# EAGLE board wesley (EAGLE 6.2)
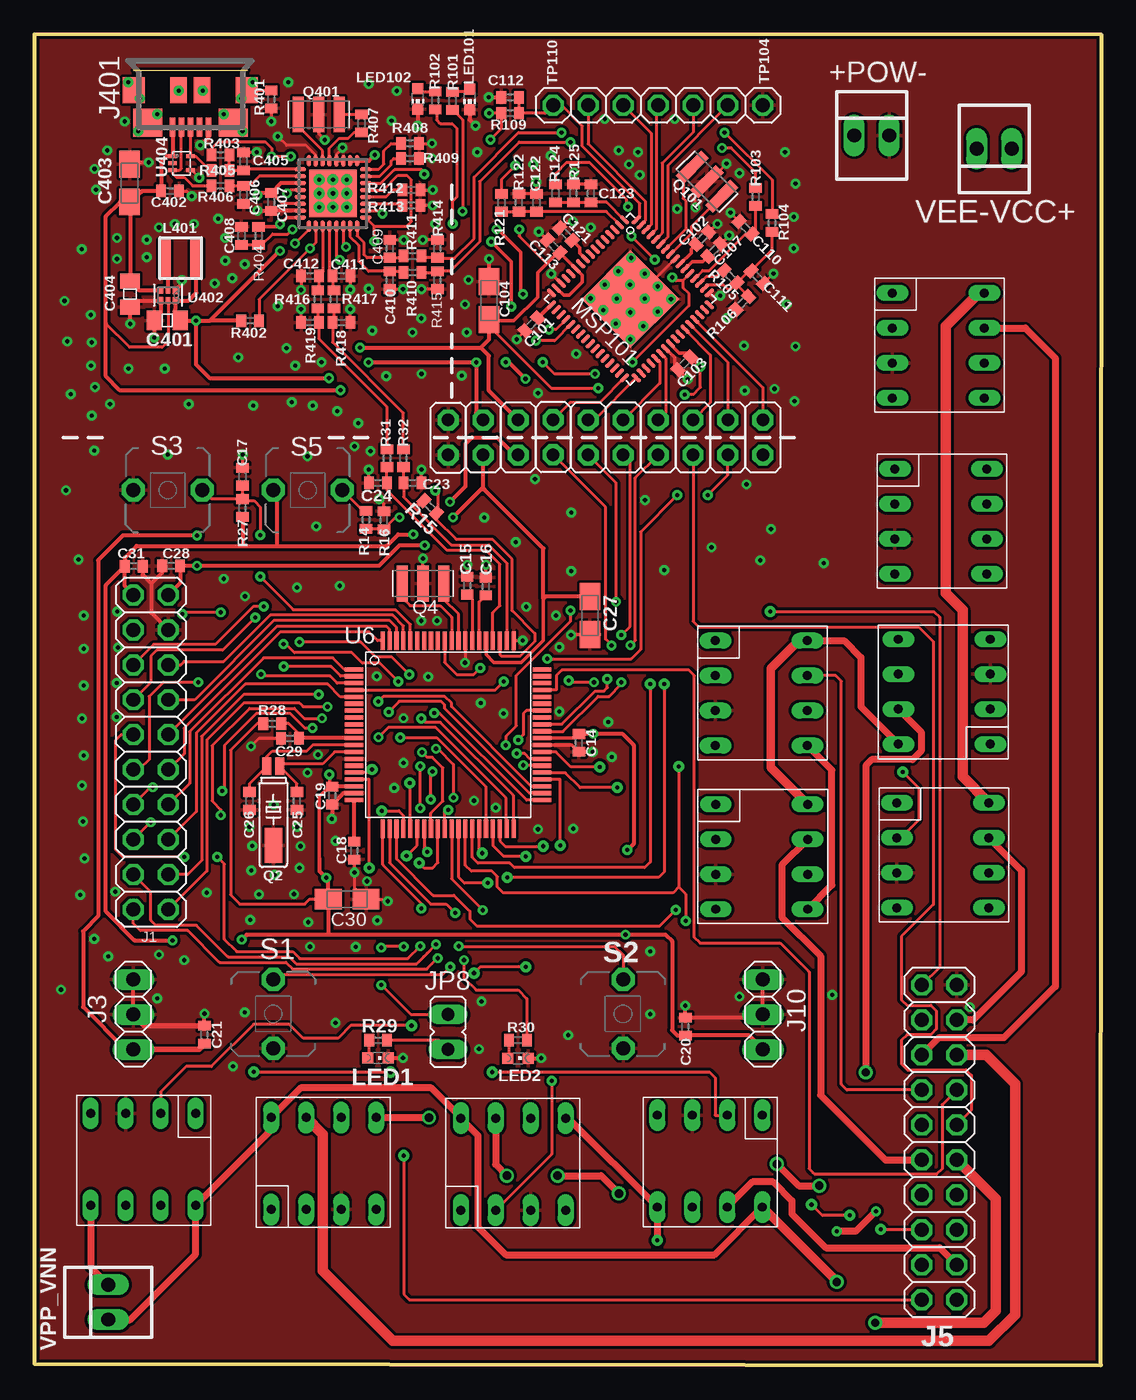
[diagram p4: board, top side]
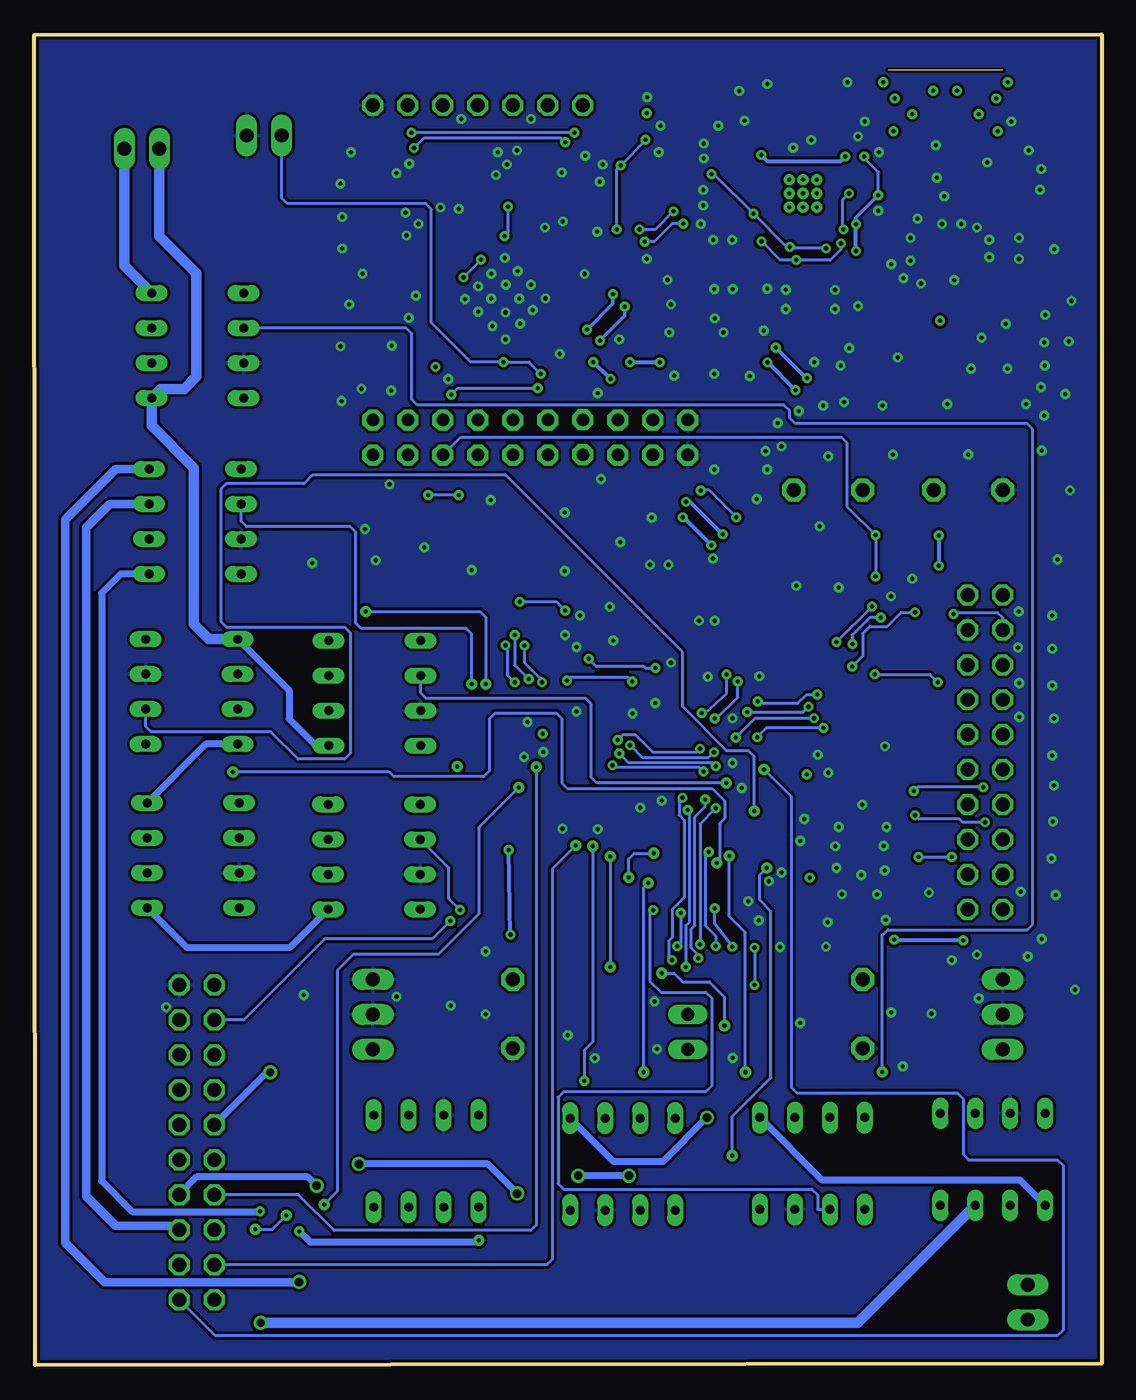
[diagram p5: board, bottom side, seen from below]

Size 77.5 x 96.67 mm. Coordinates in mm from the lower left corner, seen from the top.
Outline: 0,96.67 0,0.1 77.44,0 77.5,96.65 0,96.67
Copper layers (1*16): Top 0.0178mm / dielectric 12mil / Bottom 0.0178mm
Design rules: minimum track width 6mil, minimum drill 12mil, track to track 6mil, track to pad 6mil, pad to pad 6mil, via to via 8mil, smd to smd 6mil, copper to edge 8mil, drill to drill 8mil, minimum pad ring 10mil, minimum via ring 8mil, stop-mask expansion 8mil, vias tented up to drill 15mil, thermal gap 8mil
Net classes: 0 Default: width 0.203 mm, drill 0.305 mm, clearance 0.152 mm; 1 Ground: width 0.203 mm, drill 0.305 mm, clearance 0.152 mm to class 0, clearance 0.152 mm; 2 Power: width 0.203 mm, drill 0.305 mm, clearance 0.152 mm to class 0, clearance 0.152 mm to class 1, clearance 0.152 mm

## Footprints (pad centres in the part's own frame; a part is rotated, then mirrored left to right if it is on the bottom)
22-23-2021 = drill 1 long: 1 -1.27,0; 2 1.27,0
C0402 = smd 0.7 x 0.9: 1 -0.65,0; 2 0.65,0
A/3216-18R = smd 1.95 x 1.5: + 1.375,0; - -1.375,0
CSMD0805 = smd 1.092 x 1.397: 1 -0.94,0; 2 0.94,0
RHB_S-PQFP-N32 = smd 0.85 x 0.3: 1 -2.375,1.75; 2 -2.375,1.25; 3 -2.375,0.75; 4 -2.375,0.25; 5 -2.375,-0.25; 6 -2.375,-0.75; 7 -2.375,-1.25; 8 -2.375,-1.75; 17 2.375,-1.75; 18 2.375,-1.25; 19 2.375,-0.75; 20 2.375,-0.25; 21 2.375,0.25; 22 2.375,0.75; 23 2.375,1.25; 24 2.375,1.75 | smd 0.3 x 0.85: 9 -1.75,-2.375; 10 -1.25,-2.375; 11 -0.75,-2.375; 12 -0.25,-2.375; 13 0.25,-2.375; 14 0.75,-2.375; 15 1.25,-2.375; 16 1.75,-2.375; 25 1.75,2.375; 26 1.25,2.375; 27 0.75,2.375; 28 0.25,2.375; 29 -0.25,2.375; 30 -0.75,2.375; 31 -1.25,2.375; 32 -1.75,2.375 | smd 3.45 x 3.45: EXP 0,0 | drill 0.3 pad 0.6: EXP@1 -1,1; EXP@2 0,1; EXP@3 1,1; EXP@4 -1,0; EXP@5 0,0; EXP@6 1,0; EXP@7 -1,-1; EXP@8 0,-1; EXP@9 1,-1
2X10 = drill 1.016 octagon: 1 -11.43,-1.27; 2 -11.43,1.27; 3 -8.89,-1.27; 4 -8.89,1.27; 5 -6.35,-1.27; 6 -6.35,1.27; 7 -3.81,-1.27; 8 -3.81,1.27; 9 -1.27,-1.27; 10 -1.27,1.27; 11 1.27,-1.27; 12 1.27,1.27; 13 3.81,-1.27; 14 3.81,1.27; 15 6.35,-1.27; 16 6.35,1.27; 17 8.89,-1.27; 18 8.89,1.27; 19 11.43,-1.27; 20 11.43,1.27
1X03 = drill 1.016 long: 1 -2.54,0; 2 0,0; 3 2.54,0
HIROSE-ZX62R-B-5P = smd 1.35 x 0.4: D+ 2.675,0; D- 2.675,-0.65; GND 2.675,1.3; NC 2.675,0.65; VBUS 2.675,-1.3 | smd 1.9 x 1.6: SHIELD1 0,4.1; SHIELD2 0,-4.1 | smd 2 x 2.1: SHIELD3 2.35,3.1; SHIELD4 2.35,-3.1 | smd 1.9 x 1.2: SHIELD5 0,0.85; SHIELD6 0,-0.85
JP1M = drill 0.914 pad 1.524 octagon: 1 0,-1.27; 2 0,1.27
JP1 = drill 0.914 long: 1 0,-1.27; 2 0,1.27
L-NR3010 = smd 0.9 x 2.7: P$1 -1.15,0; P$2 1.15,0
CHIPLED_0603@1 = smd 0.8 x 0.8: A 0,-0.75; C 0,0.75
CHIP-LED0603 = smd 0.8 x 0.8: A 0,-0.75; C 0,0.75
RGC64 = smd 0.825 x 0.28: 1 -4.36,3.75; 2 -4.36,3.25; 3 -4.36,2.75; 4 -4.36,2.25; 5 -4.36,1.75; 6 -4.36,1.25; 7 -4.36,0.75; 8 -4.36,0.25; 9 -4.36,-0.25; 10 -4.36,-0.75; 11 -4.36,-1.25; 12 -4.36,-1.75; 13 -4.36,-2.25; 14 -4.36,-2.75; 15 -4.36,-3.25; 16 -4.36,-3.75; 33 4.36,-3.75; 34 4.36,-3.25; 35 4.36,-2.75; 36 4.36,-2.25; 37 4.36,-1.75; 38 4.36,-1.25; 39 4.36,-0.75; 40 4.36,-0.25; 41 4.36,0.25; 42 4.36,0.75; 43 4.36,1.25; 44 4.36,1.75; 45 4.36,2.25; 46 4.36,2.75; 47 4.36,3.25; 48 4.36,3.75 | smd 0.28 x 0.825: 17 -3.75,-4.36; 18 -3.25,-4.36; 19 -2.75,-4.36; 20 -2.25,-4.36; 21 -1.75,-4.36; 22 -1.25,-4.36; 23 -0.75,-4.36; 24 -0.25,-4.36; 25 0.25,-4.36; 26 0.75,-4.36; 27 1.25,-4.36; 28 1.75,-4.36; 29 2.25,-4.36; 30 2.75,-4.36; 31 3.25,-4.36; 32 3.75,-4.36; 49 3.75,4.36; 50 3.25,4.36; 51 2.75,4.36; 52 2.25,4.36; 53 1.75,4.36; 54 1.25,4.36; 55 0.75,4.36; 56 0.25,4.36; 57 -0.25,4.36; 58 -0.75,4.36; 59 -1.25,4.36; 60 -1.75,4.36; 61 -2.25,4.36; 62 -2.75,4.36; 63 -3.25,4.36; 64 -3.75,4.36 | smd 5 x 5: TP 0,0
8-DIP = drill 0.65 long: 1 3.81,3.81; 2 1.27,3.81; 3 -1.27,3.81; 4 -3.81,3.81; 5 -3.81,-2.87; 6 -1.27,-2.87; 7 1.27,-2.87; 8 3.81,-2.87
MS3V-T1R = smd 0.635 x 1.27: P1 -0.47,-4.43; P2 0.47,-4.43 | smd 1.27 x 2.54: P3 0,1.3
MURATA-FILTER_CSTCR = smd 0.8 x 2.6: 1 -1.5,0; 2 0,0; 3 1.5,0
R0402 = smd 0.7 x 0.9: 1 -0.65,0; 2 0.65,0
PBTH = drill 1.016 pad 1.676 octagon: 1 -0.001,0.001; 2 5.001,0.001
1X01 = drill 1.016 octagon: 1 0,0
PN80 = smd 1.35 x 0.3: 1 -6.825,4.75; 2 -6.825,4.25; 3 -6.825,3.75; 4 -6.825,3.25; 5 -6.825,2.75; 6 -6.825,2.25; 7 -6.825,1.75; 8 -6.825,1.25; 9 -6.825,0.75; 10 -6.825,0.25; 11 -6.825,-0.25; 12 -6.825,-0.75; 13 -6.825,-1.25; 14 -6.825,-1.75; 15 -6.825,-2.25; 16 -6.825,-2.75; 17 -6.825,-3.25; 18 -6.825,-3.75; 19 -6.825,-4.25; 20 -6.825,-4.75; 41 6.825,-4.75; 42 6.825,-4.25; 43 6.825,-3.75; 44 6.825,-3.25; 45 6.825,-2.75; 46 6.825,-2.25; 47 6.825,-1.75; 48 6.825,-1.25; 49 6.825,-0.75; 50 6.825,-0.25; 51 6.825,0.25; 52 6.825,0.75; 53 6.825,1.25; 54 6.825,1.75; 55 6.825,2.25; 56 6.825,2.75; 57 6.825,3.25; 58 6.825,3.75; 59 6.825,4.25; 60 6.825,4.75 | smd 0.3 x 1.35: 21 -4.75,-6.825; 22 -4.25,-6.825; 23 -3.75,-6.825; 24 -3.25,-6.825; 25 -2.75,-6.825; 26 -2.25,-6.825; 27 -1.75,-6.825; 28 -1.25,-6.825; 29 -0.75,-6.825; 30 -0.25,-6.825; 31 0.25,-6.825; 32 0.75,-6.825; 33 1.25,-6.825; 34 1.75,-6.825; 35 2.25,-6.825; 36 2.75,-6.825; 37 3.25,-6.825; 38 3.75,-6.825; 39 4.25,-6.825; 40 4.75,-6.825; 61 4.75,6.825; 62 4.25,6.825; 63 3.75,6.825; 64 3.25,6.825; 65 2.75,6.825; 66 2.25,6.825; 67 1.75,6.825; 68 1.25,6.825; 69 0.75,6.825; 70 0.25,6.825; 71 -0.25,6.825; 72 -0.75,6.825; 73 -1.25,6.825; 74 -1.75,6.825; 75 -2.25,6.825; 76 -2.75,6.825; 77 -3.25,6.825; 78 -3.75,6.825; 79 -4.25,6.825; 80 -4.75,6.825
DRY6 = smd 0.559 x 0.305: 1 -0.356,0.508 | smd 0.508 x 0.305: 2 -0.381,0; 3 -0.381,-0.508; 4 0.381,-0.508; 5 0.381,0; 6 0.381,0.508
TPD2E001-DRL = smd 0.3 x 0.6: 1 -0.5,-0.65; 2 0,-0.65; 3 0.5,-0.65; 4 0.5,0.65; 5 -0.5,0.65

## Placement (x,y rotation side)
+POW-  22-23-2021  [22-23-2021]  60.81,89.33 0 top
C14  100n  [C0402]  39.54,45.2 270 top
C15  220n  [C0402]  31.43,56.63 90 top
C16  220n  [C0402]  32.78,56.57 90 top
C17  1n  [C0402]  15.11,64.54 90 top
C18  470n  [C0402]  23.23,37.38 90 top
C19  100n  [C0402]  21.63,41.38 90 top
C20  100n  [C0402]  47.27,24.59 90 top
C21  100n  [C0402]  12.34,24 90 top
C23  10p  [C0402]  27.46,64.08 0 top
C24  10p  [C0402]  24.94,64.08 180 top
C25  12p  [C0402]  19.06,40.98 90 top
C26  12p  [C0402]  15.62,40.98 90 top
C27  4u7  [A/3216-18R]  40.34,54.46 90 top
C28  100n  [C0402]  9.93,58.06 0 top
C29  100n  [C0402]  18.57,45.53 180 top
C30  10u  [A/3216-18R]  22.71,33.85 180 top
C31  100n  [C0402]  7.21,58.04 180 top
C101  470n  [C0402]  36.09,75.61 225 top
C102  220n  [C0402]  48.5,81.86 45 top
C103  100n  [C0402]  47.21,72.77 225 top
C104  10u  [A/3216-18R]  33,77.33 270 top
C107  220n  [C0402]  49.36,81 45 top
C110  10p  [C0402]  51.64,82.63 135 top
C111  10p  [C0402]  52.5,79.04 315 top
C112  1n  [C0402]  34.55,92.09 180 top
C113  100n  [C0402]  37.7,81.27 135 top
C121  100n  [C0402]  38.6,82.17 135 top
C122  33p  [C0402]  36.46,84.45 270 top
C123  33p  [C0402]  40.41,85.13 270 top
C401  1u  [CSMD0805]  9.65,75.9 0 top
C402  100n  [C0402]  9.86,85.29 0 top
C403  4u7  [A/3216-18R]  6.91,85.88 270 top
C404  1u  [CSMD0805]  6.95,77.8 90 top
C405  22p  [C0402]  15.19,87.45 90 top
C406  22p  [C0402]  15.19,85.01 270 top
C407  100n  [C0402]  17.2,84.51 270 top
C408  100n  [C0402]  15.04,82.04 90 top
C409  22p  [C0402]  25.81,81.1 90 top
C410  22p  [C0402]  25.81,78.82 270 top
C411  22p  [C0402]  22.3,79.12 0 top
C412  22p  [C0402]  20.02,79.12 180 top
IC401  TUSB2046BIRHBIRHB  [RHB_S-PQFP-N32]  21.68,85.12 0 top
J1  [2X10]  8.46,44.53 270 top
J3  PWR  [1X03]  7.19,25.48 270 top
J5  [2X10]  65.71,16.18 270 top
J10  PWR  [1X03]  52.91,25.48 270 top
J401  [HIROSE-ZX62R-B-5P]  11.33,92.61 270 top
JP1  +5V  [JP1M]  32.59,67.39 180 top
JP2  +3V3  [JP1M]  35.13,67.39 180 top
JP3  GND  [JP1M]  30.05,67.39 0 top
JP4.1  SBW_TST  [JP1M]  50.37,67.39 180 top
JP4.2  SBW_RST  [JP1M]  47.83,67.39 180 top
JP4.3  SBW_NC  [JP1M]  52.91,67.39 180 top
JP6.1  TXD  [JP1M]  45.29,67.39 180 top
JP6.2  RXD  [JP1M]  42.75,67.39 180 top
JP6.3  CTS  [JP1M]  40.21,67.39 180 top
JP6.4  RTS  [JP1M]  37.67,67.41 180 top
JP8  LED1_PWR  [JP1]  30.05,24.21 180 top
L401  2.2uH (NR3010T2R2M)  [L-NR3010]  10.62,80.42 0 top
LED1  [CHIPLED_0603@1]  24.96,22.31 270 top
LED2  [CHIPLED_0603@1]  35.13,22.29 270 top
LED101  red  [CHIP-LED0603]  31.61,91.95 180 top
LED102  green  [CHIP-LED0603]  27.85,91.97 180 top
MSP101  MSP430F5528IRGC  [RGC64]  43.28,77.46 315 top
OPTO1  VO3150A  [8-DIP]  53.29,36.93 90 top
OPTO2  VO3150A  [8-DIP]  65.61,48.92 270 top
OPTO3  VO3150A  [8-DIP]  53.26,48.82 90 top
OPTO4  VO3150A  [8-DIP]  66.12,74.07 90 top
OPTO5  VO3150A  [8-DIP]  66.45,37.03 90 top
OPTO6  VO3150A  [8-DIP]  21.01,15.11 180 top
OPTO7  VO3150A  [8-DIP]  7.9,14.48 0 top
OPTO8  VO3150A  [8-DIP]  34.77,15.06 180 top
OPTO9  VO3150A  [8-DIP]  66.29,61.29 90 top
OPTO10  VO3150A  [8-DIP]  49.05,14.35 0 top
Q2  32.768kHz  [MS3V-T1R]  17.35,39.07 180 top
Q4  CSTCR4M00G15L99  [MURATA-FILTER_CSTCR]  28.22,56.78 0 top
Q101  PIEZO_CSTCR4M00G15L99  [MURATA-FILTER_CSTCR]  48.84,85.98 135 top
Q401  CSTCR6M00G15L99  [MURATA-FILTER_CSTCR]  20.65,90.86 0 top
R14  100R  [R0402]  24.08,61.4 270 top
R15  1k4  [R0402]  28.74,62.34 135 top
R16  1M  [R0402]  25.37,61.38 270 top
R27  47k  [R0402]  15.1,62.27 270 top
R28  0R  [R0402]  17.27,46.6 180 top
R29  470R  [R0402]  24.97,23.6 180 top
R30  470R  [R0402]  35.12,23.61 180 top
R31  27R  [R0402]  25.6,65.89 270 top
R32  27R  [R0402]  26.8,65.89 270 top
R101  470  [R0402]  30.37,91.85 270 top
R102  390  [R0402]  29.11,91.87 270 top
R103  27R  [R0402]  52.37,84.86 270 top
R104  27R  [R0402]  53.57,82.98 270 top
R105  1k4  [R0402]  50.55,79.07 135 top
R106  1M  [R0402]  51.41,77.17 45 top
R109  47k  [R0402]  34.55,90.94 180 top
R121  220k  [R0402]  33.92,84.44 270 top
R122  220k  [R0402]  35.18,84.44 90 top
R124  240k  [R0402]  37.85,85.13 270 top
R125  150k  [R0402]  39.14,85.13 90 top
R401  33R  [R0402]  17.2,91.95 270 top
R402  10k  [R0402]  15.67,75.87 0 top
R403  1k5  [R0402]  13.51,87.91 0 top
R404  47k  [R0402]  16.28,82.04 270 top
R405  22R  [R0402]  13.51,86.79 180 top
R406  22R  [R0402]  13.51,85.67 180 top
R407  1k5  [R0402]  23.75,90.2 270 top
R408  15k  [R0402]  27.28,88.75 180 top
R409  15k  [R0402]  27.28,87.66 180 top
R410  22R  [R0402]  27.46,79.38 0 top
R411  22R  [R0402]  27.46,80.57 0 top
R412  15k  [R0402]  27.38,85.37 180 top
R413  15k  [R0402]  27.38,84.25 180 top
R414  15k  [R0402]  29.26,81.1 90 top
R415  15k  [R0402]  29.26,78.82 270 top
R416  22R  [R0402]  20.57,77.42 270 top
R417  22R  [R0402]  21.74,77.42 270 top
R418  15k  [R0402]  22.3,75.74 0 top
R419  15k  [R0402]  20.02,75.74 180 top
S1  [PBTH]  17.35,28.02 270 top
S2  [PBTH]  42.75,28.02 270 top
S3  RST  [PBTH]  7.19,63.58 0 top
S5  BSL  [PBTH]  17.35,63.58 0 top
TP104  TEST_PIN2  [1X01]  52.91,91.52 0 top
TP105  TEST_PIN2  [1X01]  50.37,91.52 0 top
TP106  TEST_PIN2  [1X01]  47.83,91.52 0 top
TP107  TEST_PIN2  [1X01]  45.29,91.52 0 top
TP108  TEST_PIN2  [1X01]  42.75,91.52 0 top
TP109  TEST_PIN2  [1X01]  40.21,91.52 0 top
TP110  TEST_PIN2  [1X01]  37.67,91.52 0 top
U6  MSP430F5529IPNR  [PN80]  30.05,45.8 0 top
U402  TPS62237DRY  [DRY6]  9.7,77.72 270 top
U404  TPD2E001DRLR  [TPD2E001-DRL]  10.68,87.31 270 top
VEE-VCC+  22-23-2021  [22-23-2021]  69.7,88.37 180 top
VPP_VNN  22-23-2021  [22-23-2021]  5.36,4.57 90 top

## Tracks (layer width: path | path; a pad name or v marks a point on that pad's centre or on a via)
!OC  (via drill 0.3 pad 0.66)
  Top 0.203: IC401.14 22.43,81.43 v22.63,81.23 | IC401.10 20.43,81.54 v20.02,81.13 16.32,77.43 R402.2 | IC401.18 25.05,83.87 v25.27,83.64 | IC401.22 25.16,85.87 26.14,86.84 28.14,86.84 28.32,86.67 v28.32,86.51
  Bottom 0.203: v20.02,81.13 22.53,81.13 v22.63,81.23 22.86,81.23 v25.27,83.64 28.14,86.51 v28.32,86.51
!PWRON  (via drill 0.3 pad 0.66)
  Top 0.203: IC401.13 21.93,80.54 v22.17,80.29 | v24.69,81.64 24.69,82.73 | 24.69,82.73 IC401.17 24.69,82.73 | IC401.21 25.32,85.37 26.39,86.44 27.05,86.44 27.38,86.11 27.38,83.08 27.03,82.73 24.69,82.73 | IC401.9 19.93,82.49 v18.92,81.48
  Bottom 0.203: v24.69,81.64 23.34,80.29 v22.17,80.29 22.15,80.26 19.71,80.26 18.92,81.05 v18.92,81.48
+3V3  (via drill 0.3, 0.3 pad 0.66)
  Top 0.203: v40.59,45.87 40.61,45.87 | R28.2 16.17,46.6 14.25,44.68 14.25,34.16 14.91,33.5 19.63,33.5 19.99,33.86 21.83,33.86 C30.+ | 21.84,31.32 21.79,31.27
  Top 0.254: U6.50 39.23,45.55 C14.1 40.57,45.85 v40.59,45.87 | C31.2 6.58,58.05 | R27.2 15.11,61.61 | 20.7,36.78 20.7,41.3 21.45,42.05 | 21.65,42.05 21.45,42.05 | 21.45,42.05 21.45,42.87 v21.41,42.9
  Top 0.305: J1.1 6.56,56.58 C31.2 5.18,56.66 5.18,32.94 7.26,30.86 v10.03,30.86 | U6.18 21.65,42.05 C19.2 | 6.58,58.05 6.58,58.67 7.42,59.51 15.11,59.51 | 15.11,59.51 17.6,59.51 | 17.6,59.51 25.58,59.51 26.42,60.35 v27.51,60.35 | 15.11,61.61 15.11,59.51 | S5.1 17.6,63.32 17.6,59.51 | v40.59,45.87 42.67,45.87 43.51,45.03 43.51,37.87 v43.05,37.41 | 21.41,31.27 21.79,31.27 v42.93,31.27 45.85,31.27 46.3,30.81 46.3,24.33 46.69,23.95 47.25,23.95 C20.1 51.91,23.94 J10.3 | 21.41,31.27 15.42,31.27 v15.06,30.91 | 20.7,36.78 20.7,35.89 v21.18,35.41 21.33,35.26 C30.+ 21.33,31.35 21.41,31.27 | v30.18,62.71 31.32,63.86 31.32,66.93 31.78,67.39 33.6,67.39 34.87,66.12 JP2.2
  Bottom 0.305: v27.51,60.35 29.87,62.71 v30.18,62.71 | v10.03,30.86 14.73,30.86 v15.06,30.91 | v42.93,31.27 v43.05,37.41
+5V  (via drill 0.3 pad 0.66)
  Top 0.254: U6.65 32.8,51.61 33.38,51.03 35.36,51.03 36.96,52.63 36.96,55.68 37.11,55.83
  Top 0.305: J1.2 10.58,56.81 C28.2 v11.81,58.06 25.02,58.06 26.52,59.56 v28.35,59.56 | 36.96,55.68 36.96,59.33 32.68,63.61 32.49,63.61 32.36,63.55 | C27.+ 37.11,55.83 | v11.81,60.27 6.43,60.27 4.62,58.47 4.62,32.61 3.53,31.52 3.53,26.01 6.6,22.94 J3.3 | 12.61,23.35 C21.1 | v30.4,61.6 32.36,63.55 | 32.36,63.55 32.59,63.78 JP1.2
  Top 0.406: J3.3 11.93,22.94 C21.1
  Bottom 0.254: 30.38,61.6 v30.4,61.6
  Bottom 0.305: v28.35,59.56 30.38,61.6 | v11.81,60.27 v11.81,58.06
AVCC
  Top 0.203: C29.1 19.22,45.86 18.47,46.61 17.94,46.61 R28.1
  Top 0.305: U6.11 19.23,45.55 C29.1
EZFET_AVBUS
  Top 0.203: R124.2 | R124.2 R125.1 | R125.1 | R125.1 C123.2 41.56,84.48 MSP101.1
EZFET_AVCCOUT2ADC
  Top 0.203: R121.2 | R121.2 R122.1 C122.2 | C122.2 36.88,83.79 | MSP101.2 41.54,83.8 C122.2
EZFET_LED0  (via drill 0.3 pad 0.66)
  Top 0.203: R101.2 31.09,90.47 v31.09,83.82 | MSP101.20 37.88,75.24 v37.36,75.24
  Top 0.254: v33.55,82.5 33.68,82.5 35.33,80.85 35.33,77.95 v35.48,77.8
  Bottom 0.203: v31.09,83.82 32.41,82.5 v33.55,82.5
  Bottom 0.254: v35.48,77.8 35.48,77.11 v37.36,75.24
EZFET_LED1  (via drill 0.3 pad 0.66)
  Top 0.203: R102.2 29.21,91.12 29.21,90.48 29.49,90.2 30.33,90.2 30.66,89.87 30.66,84.84 30.38,84.56 v30.38,82.93 | MSP101.21 37.77,74.42 v36.42,74.42
  Top 0.254: v34.62,76.89 34.62,80.16 v33.17,81.61
  Bottom 0.203: v33.17,81.61 32.49,81.61 31.17,82.93 v30.38,82.93
  Bottom 0.254: v36.42,74.42 34.62,76.23 v34.62,76.89
EZFET_PU.0/DP
  Top 0.203: MSP101.50 48.91,78.49 50.04,78.49 50.34,78.18 50.57,78.18 R105.1 | R105.1 51.9,79.5 C111.1 53.57,81.03 R104.2 | R106.2 51.01,78.49 R105.1
EZFET_PU.1/DM
  Top 0.203: MSP101.52 48.53,79.53 49,79.53 51.64,82.17 C110.1 52.38,82.44 R103.2
EZFET_PUR
  Top 0.203: MSP101.51 48.81,79.1 49.56,79.1 49.99,79.53 R105.2
EZFET_RST
  Top 0.203: MSP101.64 43.97,83.45 43.97,84.38 39.8,88.54 39.8,90.02 38.3,91.52 TP110.1 37.1,90.95 R109.1 C112.1
EZFET_SBW_NC
  Top 0.203: MSP101.45 52.91,71.02 JP4.3.1
EZFET_SBW_RST
  Top 0.203: MSP101.43 47.25,75.23 49.1,73.38 49.1,69.93 JP4.2.1
EZFET_SBW_TST
  Top 0.203: MSP101.44 50.37,72.85 JP4.1.1
EZFET_TCK
  Top 0.203: MSP101.63 44.37,83.15 44.37,84.56 40.21,88.72 TP109.1
EZFET_TDI
  Top 0.203: MSP101.61 45.19,82.54 45.19,91.41 TP107.1
EZFET_TDO
  Top 0.203: MSP101.60 45.59,82.24 45.59,87.33 47.83,89.56 TP106.1
EZFET_TEST
  Top 0.203: MSP101.59 46,81.94 46,87.15 TP105.1
EZFET_TMS
  Top 0.203: MSP101.62 44.78,82.85 44.78,89.48 TP108.1
EZFET_UARTCTS
  Top 0.203: MSP101.32 41.05,69.93 38.91,69.93 JP6.4.1
EZFET_UARTRTS
  Top 0.203: MSP101.33 40.65,68.66 JP6.3.1
EZFET_UARTRXD
  Top 0.203: MSP101.38 45.51,73.49 45.85,73.15 45.85,69.22 JP6.1.1
EZFET_UARTTXD
  Top 0.203: MSP101.37 45.42,72.85 45.42,71.32 JP6.2.1
EZFET_V18
  Top 0.254: MSP101.55 46.91,80.01 47.7,80.8 47.7,81.06 C102.1
EZFET_VBUS  (via drill 0.3 pad 0.66)
  Top 0.203: R124.1 37.85,86.56 38.66,87.38 40.31,87.38 42.98,84.71 42.98,84.28 v43.1,84.15 | MSP101.53 47.6,79.28 47.09,78.77 | 47.09,78.77 46.58,78.77 v46.33,79.02 | v43.36,82.02 v45.06,80.32 | 47.09,78.77 47.09,78.28 47.55,77.83 47.55,76.96 47.52,76.96 v43.43,72.87 | v40.72,72.01 37.77,72.01 v36.91,72.87 | J401.VBUS | 9.7,75.01 U402.5 9.7,74.37 9.27,73.94 6.91,73.94 5.18,75.67
  Top 0.305: v22.23,70.84 6.17,70.84 5.18,71.83 5.18,75.67 5.18,83.46 6.22,84.5 C403.+ | v24.26,72.85 v32.08,72.85 32.08,69.16 JP1.1 | v34.24,72.87 34.44,72.87 v35.66,71.65 | C403.+ 7.83,85.29 C402.1 9.2,85.43 9.2,87.4 9.61,87.81 U404.1 J401.VBUS | U402.3 7.58,78.11 C404.2 6.95,84.46 C403.+
  Bottom 0.203: v43.1,84.15 43.1,82.3 43.36,82.04 | 43.36,82.04 v43.36,82.02 | 45.06,80.29 v45.06,80.32 46.33,79.05 v46.33,79.02 | v40.72,72.01 41.58,72.87 v43.43,72.87 45.82,72.87 48.67,75.72 48.67,83.97 49.07,84.38 59.13,84.38 59.54,84.79 +POW-.1 | 43.33,82.04 43.36,82.04
  Bottom 0.305: v22.23,70.84 24.23,72.85 v24.26,72.85 | v35.66,71.65 35.69,71.65 v36.91,72.87 | v34.24,72.87 32.08,72.87 v32.08,72.85
EZFET_VCC  (via drill 0.3 pad 0.66)
  Top 0.203: v33.02,90.96 33.89,90.96 R109.2 33.9,89.81 v33.12,89.03 | v47.22,70.51 47.83,70.51 48.36,71.04 v48.36,72.52 | C104.+ 33.06,75.45 37.54,70.97 v40.95,70.97 | R121.1 33.92,86.14 v34.93,87.15 | v35.2,82.5 35.2,82.02 37.21,80.01 | v18.62,87.81 v17.22,87.81 17.22,88.42 16.76,88.87 13.34,88.87 12.86,88.4 R403.1 | IC401.6 17.99,84.37 C407.1
  Top 0.254: MSP101.15 37.91,78.24 38.43,77.72 38.84,77.72 39.78,78.66 39.78,79.19 MSP101.11 C113.1 38.01,80.81 37.21,80.01 36.55,79.35 36.55,77.6 34.82,75.87 33.09,75.87 C104.+ | v48.36,72.52 47.67,73.21 C103.1 47.36,73.53 46.84,73.53 46.19,74.18 MSP101.40 | IC401.8 18.32,83.37 v17.83,82.88 17.64,82.69 R404.1
  Top 0.305: 21.37,71.69 v21.39,71.7 12.73,71.7 11.74,72.7 v11.74,75.87 | v23.65,73.91 32.41,73.91 | C104.+ 33,74.5 32.41,73.91 | 32.41,73.91 33,73.32 33,70.78 JP2.1 | L401.P$2 11.77,77.91 11.2,77.34 U402.6 10.21,76.68 10.21,76.28 C401.2 10.62,75.87 v11.74,75.87 | IC401.25 IC401.26 24.3,87.49 v24.71,87.91 | v11.74,75.87 12.75,75.87 | 12.75,75.87 v17.83,80.95 | IC401.3 17.91,85.87 C407.1 16.37,85.16 v16.21,84.99 | R402.1 12.75,75.87
  Bottom 0.203: v47.22,70.51 46.76,70.97 v40.95,70.97 | v33.12,89.03 33.12,88.95 v34.93,87.15 35.2,86.87 v35.2,82.5 | v16.21,84.99 16.21,86.67 17.22,87.68 v17.22,87.81
  Bottom 0.254: v17.83,82.88 17.83,83.36 v16.21,84.99
  Bottom 0.305: v21.39,71.7 21.44,71.7 v23.65,73.91 | v24.71,87.91 24.28,87.48 18.95,87.48 v18.62,87.81 | v17.83,80.95 v17.83,82.88
EZFET_VREF
  Top 0.254: MSP101.9 39.6,80.8 39.6,81.17 C121.1
EZFET_VUSB
  Top 0.254: MSP101.54 47.27,79.66 47.78,80.16 48.53,80.16 C107.1
EZFET_XT2IN
  Top 0.203: MSP101.57 47.73,82.25 47.73,82.74 Q101.1
EZFET_XT2OUT
  Top 0.203: MSP101.58 47.32,82.55 47.32,84.56 47.12,84.76 47.12,86.37 Q101.3
GND  (via drill 0.3 pad 0.66)
  Top 0.203: C405.2 15.99,88.1 v16.15,88.11 | C412.2 v19.37,78.12 v19.36,78.11 | C411.2 22.95,78.15 v22.94,78.13 | R418.2 22.95,76.69 v22.94,76.71 | R419.2 19.37,76.62 v19.36,76.71 | U6.61 v35.46,52.63 | C16.2 32.82,57.25 v32.79,58.14 | C15.2 31.45,57.29 v31.45,58.14 | U6.68 31.3,51.06 v31.27,51.03 | Q4.2 v28.22,58.6 | C24.2 24.29,64.81 v24.28,65.05 | C23.2 28.11,64.81 v28.12,65.05 | R16.1 25.37,62.59 v25.04,62.92 | C17.2 15.14,65.22 v15.14,66.14 | C18.1 23.23,35.98 v23.24,35.79 23.24,34.69 C30.- 25.51,33.85 v25.65,33.71 | C110.2 50.67,83.59 v50.55,83.72 | C111.2 53.59,79.22 v53.67,79.3 | MSP101.49 49.21,77.7 v49.81,77.7 | R106.1 v50.32,76.07 | 38.23,82.63 38.68,83.08 v39.12,83.08 | C123.1 R125.2 39.19,85.83 v39.19,86.64 | 35.2,85.12 R122.2 C122.1 36.47,85.89 v36.45,85.98 | C101.2 35.03,74.55 v35.03,74.52 | MSP101.56 44.91,78.74 | v50.27,87.27 48.97,85.98 Q101.2 48.01,85.14 v48.01,84.1 | R408.1 v28.88,88.75 | R409.1 v28.88,87.66 | R413.1 v28.93,84.25 | R412.1 v28.93,85.37 | C409.2 26.81,81.75 v26.82,81.74 | R414.2 28.21,81.75 v28.19,81.74 | R415.2 v28.13,78.17 v28.12,78.16 | C410.2 v26.76,78.17 v26.77,78.16 | R401.2 v17.2,90.35 | IC401.27 IC401.28 21.93,87.94 v22.38,88.44 | Q401.2 20.65,89.48 v21.08,89 | C29.2 16.29,45.53 v15.72,44.96 | C402.2 11.05,85.29 v11.43,84.91 | IC401.31 20.43,87.9 19.71,88.62 18.31,88.62 v17.68,89.26 | 11.38,86.81 11.41,86.81 v11.96,86.26
  Top 0.254: MSP101.14 38.25,78.61 v37.54,79.27 | C121.2 38.23,82.63 | C113.2 37.24,81.76 v36.63,82.35 | v47.45,71.63 46.76,72.31 C103.2 46.51,72.55 46.51,73.18 MSP101.39 | C107.2 49.86,81.46 v50.47,82.07 | C102.2 49.02,82.32 v49.61,82.91 | C27.- 39.01,53.08 v38.96,53.04 | U6.49 39.04,45.05 C14.2 40.51,44.55 v40.54,44.55
  Top 0.305: U404.4 11.38,86.81 | J401.GND 12.63,89.18 v12.04,88.62 | C403.- 7.03,87.38 v8.31,87.38 | U402.1 10.67,78.54 v10.69,78.82 | v8.71,74.65 C401.1 9.2,76.38 U402.4 7.43,77.34 C404.1 6.96,76.85 v6.96,75.64 | C104.- 33.02,78.22 v33.02,80.37 | LED102.C v27.85,90.05 v27.84,90.04 | LED101.C 31.61,90.46 v32.03,90.04 | C112.2 v33,92.09 v32.99,92.1 | C31.1 7.86,57.41 8.48,56.79 | 8.48,56.79 8.48,54.66 J1.4 | C28.1 9.28,57.59 8.48,56.79 | J10.1 J10.2 52.67,25.24 C20.2 v47.27,26.11 | C21.2 v12.34,25.53 | J3.2 J3.1 | LED1.C 26.76,22.31 v26.77,22.33 | LED2.C 36.77,22.29 36.78,22.3 v36.8,22.3 | U6.19 22.45,41.55 C19.1 21.63,39.71 v21.59,39.68 | v16.21,83.87 C407.2 IC401.7 | v45.26,78.36 45.03,78.36 44.37,79.02 44.63,79.02 44.91,78.74
  Top 0.406: C21.2 8.01,24.65 J3.2
  other vias: 19.08,39.09 15.62,39.09 43.33,80.44 40.39,77.5 42.21,75.67 46.23,77.44 44.32,79.3 42.39,79.48 41.43,78.49 43.26,78.49 42.29,77.47 41.3,76.63 43.28,74.52 44.22,75.49 45.26,76.53 44.32,77.47 43.28,76.48 46.69,84 3.2,58.52 2.29,63.55 4.17,68.99 9.68,66.14 19.84,66.01 20.47,60.93 15.29,55.85 19.08,56.49 22.17,56.62 29.24,54.08 24.87,50.04 28.6,50.01 26.8,46.99 41.94,44.17 34.06,47.35 35.71,55.09 32.66,61.57 36.35,64.36 67.92,26.01 52.71,58.47 38.13,52.17 38.99,61.93 38.99,57.68 45.75,57.76 44.35,62.84 51.71,63.98 49.17,59.41 55.19,70.03 51.54,74.07 55.27,74.02 54.64,77.06 55.14,81.13 55.27,85.83 54.51,88.11 55.14,83.41 51.21,86.59 43.97,86.46 43.84,88.11 42.44,88.24 37.49,87.86 36.22,87.22 40.41,82.65 43.18,87.22 41.43,90.53 46.51,90.53 26.31,92.56 25.93,90.4 29.11,82.91 31.27,77.06 32.16,88.11 31.52,78.84 27.46,75.03 28.09,76.05 24.28,78.21 24.54,75.16 28.12,72.01 25.55,71.86 51.59,70.79 22,69.32 23.52,68.43 31.39,75.03 24.41,66.4 23.24,66.75 20.22,69.7 18.69,69.95 18.95,72.62 20.85,72.87 18.31,73.89 17.68,76.94 15.27,79.98 14.38,78.97 13.11,78.59 13.87,80.24 13.87,81.89 13.36,83.29 11.58,82.91 10.19,82.91 9.04,82.65 8.15,81.76 8.15,80.49 24.28,93.07 18.44,93.19 5.99,81.89 5.99,80.37 6.55,90.35 2.39,74.37 2.18,77.32 5.28,88.24 4.37,86.89 2.64,70.54 3.43,81.08 4.47,85.39 4.09,76.3 4.17,74.3 4.11,72.62 4.39,71.04 5.49,69.82 11.2,69.82 15.9,69.7 3.58,54.46 4.34,66.45 3.58,52.04 3.58,49.38 3.45,46.96 3.58,44.3 3.45,42.11 3.53,39.5 3.63,36.8 3.33,34.16 4.34,30.96 5.36,29.69 10.87,29.41 23.34,30.38 51.21,26.77 38.13,47.47 41.68,46.71 39.14,38.96 32.41,48.11 31.93,41 53.49,60.73 24.89,32.31 33.5,40.49 26.14,41.94 26.8,43.74 36.58,38.94 21.87,38.07 24.16,35.15 18.85,34.21 21.87,24.87 14.43,21.69 32.28,22.96 38.76,23.98 32.46,26.42 44.73,25.5 13.74,57.12 57.94,26.9 1.93,27.28 17.45,35.61 15.75,35.94 19.25,36.12 19.33,37.69 17.37,40.72 15.82,37.72 19.84,43.03 28.09,54.08 6.07,52.12 34.95,59.79 37.87,54.46 20.02,30.4 44.73,30.05 36.58,70.61 39.34,73.46 53.75,70.92 31.04,71.88 57.33,58.27 6.02,54.74 5.97,49.56 5.97,47.09 15.67,32.33 12.52,34.32 5.87,34.39 20.6,44.35 16.31,34.19 19.89,32.18 6.83,72.39 9.47,72.39 14.81,73.2 8.92,26.64 15.27,25.63 9.04,29.82
  pour Top (isolate 0.203, rank 2): -1.96,98.53 -1.83,-1.32 78.94,-1.85 78.69,98.35
  pour Bottom (isolate 0.203, rank 2): -2.41,98.93 -1.93,-1.7 79.1,-1.4 78.82,98.53
  pour Top (isolate 0.203): 24.23,45.54 15.44,45.54 14.66,44.78 14.63,35.92 15.54,34.95 19.28,34.95 20.22,35.86 20.22,42.67 21.59,44.04 24.23,44.04
  pour Top (isolate 0.203): 23.27,92.07 22.5,92.84 18.92,92.84 18.26,92.18 18.26,89.38 20.02,87.07 22.48,87.02 22.91,88.47 22.91,88.67 24.49,88.67 24.49,92.13
  pour Top (isolate 0.203): 31.32,51.64 31.34,54.94 30.76,55.52 30.73,58.06 29.97,58.83 26.39,58.83 25.73,58.17 25.73,55.37 26.47,54.64 29.46,54.64 29.77,54.33 29.77,51.64
HUB_DM1
  Top 0.203: R416.2 20.57,75.83 R419.1 20.67,74.56 25.6,69.62 R31.1
HUB_DM2  (via drill 0.3 pad 0.66)
  Top 0.203: R103.1 52.4,85.54 52.4,86.64 50.62,88.42 v49.94,88.42 | v38.94,88.85 35.2,88.85 32.33,85.98 32.33,81.61 30.19,79.47 R415.1 29.17,79.38 R410.2
  Bottom 0.203: v49.94,88.42 49.23,89.13 39.22,89.13 v38.94,88.85
HUB_DP1
  Top 0.203: R417.2 21.74,75.83 R418.1 21.65,74.31 26.8,69.16 R32.1
HUB_DP2  (via drill 0.3 pad 0.66)
  Top 0.203: R104.1 53.57,86.11 50.14,89.54 v50.11,89.54 | v38.28,89.54 35.15,89.54 31.93,86.31 31.93,81.84 30.51,80.42 29.3,80.42 R414.1 28.22,80.45 R411.2
  Bottom 0.203: v38.28,89.54 v50.11,89.54
N$1
  Top 0.203: 30.41,92.45 R101.1 31.41,92.5 LED101.A
N$2
  Top 0.203: LED102.A 27.9,92.52 R102.1
N$3
  Top 0.203: IC401.15 22.91,82.72 22.91,81.99 23.55,81.36 23.55,80.19 24.27,79.47 C410.1 26.72,79.47 R410.1
N$4
  Top 0.203: R14.1 23.87,62.05 S5.2
N$5
  Top 0.203: R403.2 R405.1 15.18,86.79 C405.1 15.25,86.87 IC401.1
N$6
  Top 0.203: IC401.30 20.93,88.22 19.15,89.99 Q401.1
N$7
  Top 0.203: R29.1 29.39,23.6 JP8.2
N$8
  Top 0.305: MSP101.17 36.57,76.05 C101.1
N$9  (via drill 0.3 pad 0.3)
  other vias: 7.54,89.64
N$10
  Top 0.203: R401.1 15.44,92.6 J401.SHIELD1
N$11
  Top 0.203: R406.1 C406.1 15.33,85.8 15.75,85.8 16.31,86.37 IC401.2
N$12
  Top 0.203: J401.D+ U404.5 11.73,87.81 12.75,86.79 R405.2
N$13
  Top 0.203: J401.D- 10.67,89.92 10.67,86.94 10.54,86.81 U404.3 10.03,86.57 10.31,86.28 10.87,86.28 11.48,85.67 R406.2
N$14
  Top 0.305: U402.2 9.7,79.3 9.47,79.53 L401.P$1
N$15
  Top 0.203: R407.2 23.2,89.55 22.78,89.13 22.15,89.13 21.43,88.41 IC401.29
N$16
  Top 0.203: IC401.11 20.93,79.39 C412.1 20.67,78.16 R416.1
N$17
  Top 0.203: IC401.12 21.43,79.34 C411.1 21.65,78.16 R417.1
N$18
  Top 0.203: IC401.16 23.44,82.73 23.44,82.04 23.95,81.53 23.95,80.67 24.17,80.45 C409.1 26.69,80.45 R411.1
N$19  (via drill 0.3 pad 0.66)
  Top 0.203: IC401.4 18.59,85.37 v18.34,85.12 | C408.1 R404.2 16.52,81.39 17.3,82.17 18.42,82.17 v18.75,82.5
  Bottom 0.203: v18.34,85.12 18.82,84.63 18.82,82.58 v18.75,82.5
N$20
  Top 0.203: R412.2 26.04,85.37 25.53,84.86 IC401.20
N$21
  Top 0.203: IC401.24 24.99,86.87 25.37,87.25 25.37,88.21 25.91,88.75 R408.2
N$22
  Top 0.203: IC401.23 25.08,86.37 25.91,87.2 25.91,87.48 26.09,87.66 R409.2
N$23
  Top 0.203: IC401.19 26.59,84.37 R413.2
N$24  (via drill 0.3 pad 0.3)
  other vias: 8.92,90.88
N$25  (via drill 0.3 pad 0.3)
  other vias: 13.74,90.88
N$26  (via drill 0.3 pad 0.3)
  other vias: 15.11,89.64
N$27  (via drill 0.3 pad 0.3)
  other vias: 15.85,93.19
N$28
  Top 0.203: R407.1 22.16,90.85 Q401.3
N$29  (via drill 0.3 pad 0.3)
  other vias: 15.01,92.02
N$30  (via drill 0.3 pad 0.3)
  other vias: 7.65,92.02
N$31  (via drill 0.3 pad 0.3)
  other vias: 6.81,93.19
N$32
  Top 0.203: LED1.A 24.32,22.43 R29.2
N$33  (via drill 0.3 pad 0.3)
  other vias: 10.49,92.58
N$34  (via drill 0.3 pad 0.3)
  other vias: 12.22,92.58
N$35
  Top 0.203: LED2.A 34.47,22.38 R30.2
P1.0  (via drill 0.3 pad 0.3)
  Top 0.203: U6.21 25.3,36.35 28.09,33.55 v28.09,33.17 | U6.21 | v25.2,27.61 27.33,25.48 JP8.1 | v26.82,30.4 25.27,30.4 v25.2,30.33
  Bottom 0.203: v25.2,30.33 v25.2,27.61 | v26.82,30.4 28.09,32.06 v28.09,33.17
P1.1  (via drill 0.3)
  Top 0.203: U6.22 25.8,36.48 28.78,33.5 29.9,33.5 v30.56,32.84 | v30.81,30.43 42.11,30.43 42.75,29.79 S2.1
  Bottom 0.203: v30.56,32.84 30.56,30.68 v30.81,30.43
P1.2  (via drill 0.3)
  Top 0.203: v46.58,33.07 45.39,31.88 32.16,31.88 31.62,32.41 31.62,32.97 30.45,34.14 28.93,34.14 26.3,36.77 U6.23
  Bottom 0.203: v46.58,33.07 47.4,33.88 47.4,36.12 OPTO1.2
P1.3  (via drill 0.3 pad 0.81)
  Top 0.203: v25.22,40.26 26.47,40.26 26.8,39.93 U6.24
  Bottom 0.203: v25.22,40.26 25.22,44.22 25.63,44.63 27.23,44.63 30.43,47.83 30.43,51.79 43.28,64.64 57.3,64.64 57.91,64.03 63.55,64.03 63.96,63.63 63.96,54.03 63.55,53.62 54.97,53.62 54.56,53.21 54.56,44.42 54.97,44.02 58.34,44.02 60.33,46 69.01,46 69.42,46.41 OPTO2.2
P1.4  (via drill 0.3 pad 0.81)
  Top 0.203: v27.25,42.29 27.25,39.41 27.3,39.37 U6.25
  Bottom 0.203: v27.25,42.29 36.65,42.29 37.06,42.7 37.06,48.03 37.47,48.44 49.05,48.44 49.45,48.84 OPTO3.2
P1.5  (via drill 0.3 pad 0.81)
  Top 0.203: v15.93,21.31 25.83,21.31 v25.86,21.29 | v27.03,36.98 27.8,37.76 U6.26
  Bottom 0.203: v25.86,21.29 25.86,31.42 27.03,32.59 v27.03,36.98 | v15.93,21.31 15.93,31.22 15.52,31.62 5.41,31.62 5,32.03 5,68 5.41,68.4 22.25,68.4 22.66,68.81 22.66,69.34 23.06,69.75 49.68,69.75 50.09,70.16 50.09,74.93 50.5,75.34 OPTO4.2
P1.6  (via drill 0.3)
  Top 0.203: U6.27 28.3,37.51 v28.52,37.29 | 27.76,30.18 v28.02,30.43 27.13,29.54 19.25,29.54 18.75,30.05 14.68,30.05 13.79,30.94 13.79,36.4 v13.28,36.91 | v10.87,36.91 6.43,36.91 5.92,37.41 5.92,45.42 6.3,45.8 J1.9
  Bottom 0.203: v13.28,36.91 v10.87,36.91 | v28.52,37.29 28.78,37.03 28.78,31.95 28.02,31.19 v28.02,30.43
P1.7  (via drill 0.3)
  Top 0.203: U6.28 28.8,40.1 29.67,40.97 29.67,43.38 28.91,44.15 28.52,44.15 v28.14,44.53 | v38.94,54.81 38.94,54.05 35,50.11 35,46.43 34.24,45.67 v34.24,45.03 | v42.24,55.45 42.24,64.08 JP6.3.2
  Bottom 0.203: v38.94,54.81 39.57,55.45 v42.24,55.45 | v28.14,44.53 28.52,44.15 33.35,44.15 v34.24,45.03
P2.0  (via drill 0.3 pad 0.81)
  Top 0.203: U6.29 29.3,36.51 28.88,36.09 28.32,36.09 v27.94,36.47 | v63.07,43.08 64.21,41.94 64.21,39.6 62.92,38.3 OPTO5.2
  Bottom 0.203: v63.07,43.08 | v27.94,36.47 27.74,36.68 27.74,39.34 27.36,39.73 27.36,40.97 28.27,41.88 38.79,41.88 39.19,42.29 39.19,46.96 39.6,47.37 44.04,47.37 44.44,46.96 44.44,43.19 44.88,42.75 51.38,42.75 51.71,43.08 v63.07,43.08
P2.1  (via drill 0.3, 0.3 pad 0.66)
  Top 0.203: U6.30 29.79,40.16 29.97,40.34 v30.05,40.34 | S1.1 17.53,28.02 17.91,28.4 29.67,28.4 v30.2,28.93
  Bottom 0.203: v30.05,40.34 29.92,40.21 29.92,32.21 30.18,31.95 30.18,28.96 v30.2,28.93
P2.2  (via drill 0.3)
  Top 0.203: U6.31 30.3,35.34 32.56,33.07 v32.56,33.05
  Bottom 0.203: OPTO6.2 20.63,11.3 20.63,12.37 21.03,12.78 39.07,12.78 39.47,13.18 39.47,19.46 39.07,19.86 28.73,19.86 28.32,20.27 28.32,26.67 28.73,27.08 31.98,27.08 32.79,27.89 32.79,32.82 v32.56,33.05
P2.3  (via drill 0.3 pad 0.81)
  Top 0.203: v32.92,35.03 31.22,35.03 30.8,35.45 U6.32 | OPTO10.2 49.43,18.16 49.43,20.88 49.02,21.29 v33.25,21.29
  Bottom 0.203: v33.25,21.29 33.25,34.7 v32.92,35.03
P2.4  (via drill 0.3, 0.3 pad 0.81)
  Top 0.203: v46.79,43.49 46.79,34.72 | 46.79,34.72 46.38,34.32 34.04,34.32 33.63,34.72 33.63,35.48 33.22,35.89 31.72,35.89 31.3,36.32 U6.33 | 46.79,34.72 47.3,34.21 v47.3,32.26
  Bottom 0.203: v47.3,32.26 48.59,30.96 56.41,30.96 62.31,25.07 J5.3
P2.5  (via drill 0.3 pad 0.81)
  Top 0.203: v44.73,49.48 44.73,36.55 44.32,36.14 34.85,36.14 34.52,36.47 32.21,36.47 31.8,36.88 U6.34 | v53.44,54.74 65.33,54.74 65.74,54.33 65.74,28.91 J5.1
  Bottom 0.203: v53.44,54.74 45.14,54.74 44.73,54.33 v44.73,49.48
P2.6  (via drill 0.3 pad 0.81)
  Top 0.203: v32.51,37.19 32.51,37.49 32.3,37.49 U6.35 | v45.75,49.48 45.75,35.84 45.34,35.43 v34.34,35.43
  Bottom 0.203: v34.34,35.43 34.34,36.78 33.93,37.19 v32.51,37.19 | v45.75,49.48 45.75,53.11 46.15,53.52 53.75,53.52 54.15,53.92 54.15,60.5 54.56,60.91 62.08,60.91 62.48,61.32 OPTO9.2
P2.7  (via drill 0.3 pad 0.66)
  Top 0.203: 32.79,38.98 U6.36 32.8,42.01 29.21,45.59 v26.57,45.59 | v13.54,39.95 13.54,40.34 12.9,41 12.9,45.01 15.62,47.7 18.87,47.7 19.58,46.99 v20.88,46.99 | v8.46,39.45 J1.15
  Bottom 0.203: v13.54,39.95 13.28,39.7 10.36,39.7 10.11,39.45 v8.46,39.45 | v20.88,46.99 25.17,46.99 v26.57,45.59
P3.0  (via drill 0.3 pad 0.81)
  Top 0.203: U6.37 33.3,37.75 34.06,36.98 35.66,36.98 v35.69,36.96 | v35.69,28.93 32.39,28.93 v31.93,28.47 | v27.38,24.66 22.96,24.66 22.05,23.75 19.53,23.75 18.52,24.77 15.93,24.77 12.85,21.69 11.02,21.69 9.17,19.84 OPTO7.2
  Bottom 0.203: v35.69,36.96 v35.69,28.93 | v31.93,28.47 31.04,28.47 30.4,27.84 28.47,27.84 27.38,26.75 v27.38,24.66
P3.1  (via drill 0.3, 0.3 pad 0.81)
  Top 0.203: U6.38 33.8,38.08 34.19,37.69 v36.96,37.69 | v37.57,20.65 37.57,15.32 OPTO8.2
  Bottom 0.203: v36.96,37.69 36.96,23.47 37.57,22.86 v37.57,20.65
P3.2  (via drill 0.3 pad 0.66)
  Top 0.203: U6.39 34.26,39.01 34.26,41.2 29.16,46.3 25.68,46.3 v24.99,45.62 | v13.64,41.71 13.79,41.86 13.79,45.01 16.1,47.32 18.59,47.32 19.63,46.28 v20.19,46.28 | v8.59,41.99 8.46,41.99 J1.13
  Bottom 0.203: v8.59,41.99 13.36,41.99 v13.64,41.71 | v20.19,46.28 24.33,46.28 v24.99,45.62
P3.3  (via drill 0.3 pad 0.3, 0.3 pad 0.66)
  Top 0.203: U6.40 34.77,39 34.77,41.4 29.49,46.69 28.37,46.69 v28.09,46.96 | v26.42,49.66 25.07,51 23.83,51 23.06,51.77 18.87,51.77 18.26,52.38 v18.09,52.38 | v16.03,54.31 13.67,51.94 8.89,51.94 8.46,51.51 8.46,49.61 J1.7
  Bottom 0.203: v26.42,49.66 26.42,48.51 27.97,46.96 v28.09,46.96 | v16.03,54.31 16.84,54.31 18.11,53.04 18.11,52.4 v18.09,52.38
P3.4  (via drill 0.3 pad 0.3, 0.3 pad 0.66)
  Top 0.203: U6.41 35.74,41.05 29.41,47.37 v29.03,47.37 | v19.25,52.53 23.7,52.53 24.79,51.44 25.96,51.44 v27.23,50.17 | v16.66,55.12 15.9,55.12 13.13,52.35 8.66,52.35 J1.5
  Bottom 0.203: v27.23,50.17 27.23,48.79 28.78,47.37 v29.03,47.37 | v19.25,52.53 v16.66,55.12
P3.5  (via drill 0.3)
  Top 0.203: U6.42 35.95,41.55 29.79,47.7 29.79,47.96 29.54,48.21 26.49,48.21 v25.73,47.45 | J1.20 12.52,35.89 12.52,45.42 15.19,48.08 19.25,48.08 19.51,47.83 v21.29,47.83
  Bottom 0.203: v25.73,47.45 21.67,47.45 v21.29,47.83
P3.6  (via drill 0.3)
  Top 0.203: U6.43 36.08,42.05 30.3,47.83 30.3,48.08 29.79,48.59 25.35,48.59 v24.97,48.21 | J1.18 11.12,35.64 12.14,36.66 12.14,45.67 15.19,48.72 v20.65,48.72
  Bottom 0.203: v24.97,48.21 24.84,48.08 22.05,48.08 21.41,48.72 v20.65,48.72
P3.7  (via drill 0.3 pad 0.81)
  Top 0.203: v38.18,37.74 38.18,42.55 U6.44
  Bottom 0.203: v38.18,37.74 39.88,36.04 39.88,7.7 40.28,7.29 J5.17
P4.0  (via drill 0.3 pad 0.81)
  Top 0.203: J5.15 61.49,9.83 v61.47,9.86 | v59.21,10.87 57.23,10.87 v56.44,11.66 | v42.32,41.96 39.62,41.96 38.56,43.03 36.89,43.03 U6.45
  Bottom 0.203: v61.47,9.86 60.22,9.86 v59.21,10.87 | v56.44,11.66 56.44,11.68 55.47,12.65 55.47,28.7 54.31,29.87 48.13,29.87 45.19,32.82 45.19,39.09 v42.32,41.96
P4.1  (via drill 0.3 pad 0.66)
  Top 0.203: v28.78,41.1 28.78,42.98 v28.91,43.13 | 28.98,29.26 v29.29,29.57 28.5,28.78 18.75,28.78 18.26,29.26 13.44,29.26 11.13,31.57 7.7,31.57 7.19,32.08 J1.19 | U6.46 35.55,43.55 v35.51,43.59
  Bottom 0.203: v28.91,43.13 29.18,43.41 35.33,43.41 v35.51,43.59 | 28.78,40.72 v28.78,41.1 28.78,40.59 29.54,39.83 29.54,31.95 29.79,31.7 29.79,30.3 29.29,29.79 v29.29,29.57
P4.2  (via drill 0.3)
  Top 0.203: J1.17 8.46,34.37 8.46,32.31 8.82,31.95 11.76,31.95 14.05,29.67 18.49,29.67 19,29.16 27.76,29.16 28.27,29.67 28.52,29.92 v29.16,30.56 | v28.02,40.46 v28.02,43.51 | U6.47 35.99,44.05 35.61,44.43 v35.03,44.43
  Bottom 0.203: v28.02,40.46 29.16,39.32 v29.16,30.56 | v28.02,43.51 28.27,43.76 34.37,43.76 v35.03,44.43
P4.3  (via drill 0.3 pad 0.81)
  Top 0.203: v41.05,43.46 38.96,43.46 37.87,44.55 U6.48
  Bottom 0.203: v41.05,43.46 41.05,10.19 41.45,9.78 55.73,9.78 58.32,12.37 J5.13
P4.4/UCA1TXD  (via drill 0.3)
  Top 0.203: U6.51 36.89,46.03 38.38,46.03 40.95,48.59 41.73,48.59 42.62,49.48 v42.62,49.61 | v43.28,52.3 43.64,52.65 43.64,64.47 JP6.1.2
  Bottom 0.203: v42.62,49.61 43.13,50.11 43.13,52.15 v43.28,52.3
P4.5/UCA1RXD  (via drill 0.3)
  Top 0.203: U6.52 36.89,46.56 38.3,46.56 40.72,48.97 41.35,48.97 41.61,49.23 v41.61,49.84 | v42.62,53.04 43.26,53.67 43.26,65.61 JP6.2.2
  Bottom 0.203: v42.62,53.04 42.62,50.85 v41.61,49.84
P4.7  (via drill 0.3)
  Top 0.203: U6.54 35.74,47.55 35.51,47.32 35.51,45.8 v35.13,45.42 | v31.19,29.41 31.19,28.14 32.08,27.25 35.13,27.25 35.76,26.62 R30.1 | v29.16,44.78 29.29,44.78 30.43,43.64 v30.43,41.22
  Bottom 0.203: v30.43,41.22 30.68,40.97 30.68,39.95 30.3,39.57 30.3,33.99 31.19,33.1 31.19,31.06 31.45,30.81 31.45,29.67 v31.19,29.41 | v29.16,44.78 29.41,44.53 32.59,44.53 33.86,45.8 34.75,45.8 v35.13,45.42
P5.2/XT2IN
  Top 0.203: U6.69 30.8,54.55 29.72,55.63 Q4.3
P5.3/XT2OUT
  Top 0.203: Q4.1 26.72,55.73 27.28,55.17 29.46,55.17 30.3,54.33 U6.70
P5.4/XIN
  Top 0.203: U6.12 20.21,45.05 19.76,44.6 17.27,44.6 16.88,44.21 Q2.P2 15.62,42.24 C26.2
P5.5/XOUT
  Top 0.203: C25.2 19.06,42.25 Q2.P1 | Q2.P1 17.87,43.5 | U6.13 21.79,44.55 20.93,43.69 18.01,43.69 Q2.P1
P6.0
  Top 0.203: U6.77 26.8,53.69 26.01,54.48 17.12,54.48 13.77,51.13 10.87,51.13 10.62,50.88 J1.6
P6.1
  Top 0.203: U6.78 26.3,53.59 25.81,54.08 17.37,54.08 11.63,48.34 J1.8
P6.2
  Top 0.203: U6.79 25.8,53.45 25.58,53.67 17.6,53.67 J1.10
P6.3
  Top 0.203: U6.80 24.93,52.62 24.28,53.26 17.86,53.26 10.87,46.28 10.87,44.4 J1.12
P6.4
  Top 0.203: J1.14 11.28,42.27 11.28,46.03 16.64,51.38 21.67,51.38 22.5,50.55 U6.1
P6.5  (via drill 0.3)
  Top 0.203: v13.54,54.69 10.87,54.69 v10.74,54.56 | U6.2 22.24,50.05 21.54,50.75 v18.11,50.75
  Bottom 0.203: v10.74,54.56 10.62,54.69 7.57,54.69 7.19,54.31 J1.3 | v13.54,54.69 14.55,54.69 15.57,53.67 16.84,53.67 17.35,53.16 17.35,51.51 v18.11,50.75
P6.6  (via drill 0.3, 0.3 pad 0.66)
  Top 0.203: v11.89,49.61 9.36,49.61 8.33,48.58 8.33,44 7.59,43.26 J1.11 | U6.3 21.98,49.55 21.47,50.05 16.59,50.05 v16.46,50.18
  Bottom 0.203: v16.46,50.18 12.46,50.18 v11.89,49.61
P6.7  (via drill 0.3 pad 0.3, 0.3 pad 0.66)
  Top 0.203: U6.4 33.48,49.05 v34.09,49.66 | v41.91,52.27 41.48,52.73 41.48,62.33 JP6.4.2 | v40.64,49.61 38.94,49.61 v38.81,49.73
  Bottom 0.203: v41.91,52.27 41.91,51.05 40.64,49.78 v40.64,49.61 | 34.09,49.63 v34.09,49.66 34.42,49.99 38.56,49.99 v38.81,49.73
P7.0
  Top 0.203: J1.16 11.76,40.21 11.76,45.92 15.32,49.48 21.29,49.48 22.22,48.55 U6.5
P7.4
  Top 0.203: J5.8 65.91,18.92 65.91,14.25 65.51,13.84 56.69,13.84 56.52,14.02 56.29,14.25 56.26,14.28 56.26,28.55 54.15,30.66 48.34,30.66 47.93,31.06 47.93,50.09 47.52,50.5 38.3,50.5 37.9,50.09 37.9,49.05 U6.57
P8.1  (via drill 0.3 pad 0.81)
  Top 0.203: v24.51,43.28 24.28,43.05 U6.16
  Bottom 0.203: v24.51,43.28 22.53,41.3 22.53,20.17 22.12,19.76 10.47,19.76 10.06,19.36 10.06,15.32 9.65,14.91 3.2,14.91 2.79,14.5 2.79,2.54 3.2,2.13 64.36,2.13 J5.20
P8.2  (via drill 0.3 pad 0.81)
  Top 0.203: v24.31,36.12 24.31,42.55 U6.17 | v26.82,15.21 26.82,5.16 27.23,4.75 J5.19
  Bottom 0.203: v26.82,15.21 26.82,18.06 24,20.88 24,32.97 24.82,33.78 24.82,35.61 v24.31,36.12
RST/SBWTDIO  (via drill 0.3 pad 0.66)
  Top 0.203: R27.1 12.85,62.92 S3.2 | U6.76 27.3,53.8 26.21,54.89 18.8,54.89 v16.41,57.28 | R27.1 15.23,62.79 15.95,62.79 16.41,62.33 v16.41,60.3 | C17.1 15.1,63.88 R27.1 | JP4.2.2 47.83,54.03 48.23,53.62 64.21,53.62 65.28,52.55 65.28,33.45 62.97,31.14 62.97,26.54 63.37,26.14 65.1,26.14 65.51,25.73 65.51,24.41 65.1,24 63.37,24 62.97,23.6 62.97,21.87 63.37,21.46 67.64,21.46 68.05,21.06 68.05,18.52 J5.10
  Bottom 0.203: v16.41,57.28 v16.41,60.3 18.49,62.38 18.49,67.01 18.9,67.41 46.53,67.41 JP4.2.2
TARGET_DM
  Top 0.203: U6.64 33.3,54.66 33.81,55.17 33.81,58.19 32.82,59.18 29.97,59.18 25.59,63.56 C24.1 R31.2
TARGET_DP
  Top 0.203: 34.26,52.66 U6.62 34.3,58.29 32.99,59.59 30.29,59.59 27.4,62.48 | R32.2 C23.1 26.81,63.07 27.4,62.48 | R15.2 27.95,62.48 27.4,62.48
TARGET_PUR  (via drill 0.3 pad 0.66)
  Top 0.203: U6.63 33.81,52.61 33.81,51.61 33.91,51.51 35.28,51.51 36.35,52.58 36.35,53.16 34.7,54.81 34.7,58.55 33.25,60 30.63,60 29.2,61.43 R15.1 | R14.2 25.35,60.75 R16.2 26.24,61.6 v26.52,61.6 | R15.1 29.13,61.95 | v29.11,63.53 29.34,63.3 29.34,62.02 R15.1
  Bottom 0.203: v26.52,61.6 28.5,63.58 29.06,63.58 v29.11,63.53
TARGET_VUSB
  Top 0.203: U6.66 32.3,55.44 C16.1
TEST/SBWTCK  (via drill 0.3, 0.3 pad 0.66)
  Top 0.203: U6.71 29.8,51.05 30.68,50.17 31.9,50.17 v32.39,50.65 | v37.24,51.31 43.33,51.31 44.02,51.99 44.02,60.53 v46.69,63.2 | v48.9,63.2 50.37,64.67 JP4.1.2
  Bottom 0.203: v37.24,51.31 36.68,50.75 33.22,50.75 33.12,50.65 v32.39,50.65 | v46.69,63.2 v48.9,63.2
V18
  Top 0.203: C15.1 31.8,55.61 U6.67
VCC+
  Top 0.508: OPTO3.8 58.8,52.63 60.02,51.41 60.02,47.83 OPTO2.8
  Top 0.635: OPTO1.8 53.47,43.43 53.47,50.6 55.5,52.63 OPTO3.8
  Top 0.762: OPTO4.8 68.58,77.88 66.19,75.49 66.19,56.08 67.41,54.86 67.41,42.75 OPTO5.8
  Bottom 0.508: OPTO2.8 65.05,45.11 OPTO5.8
  Bottom 0.762: VEE-VCC+.1 70.97,79.86 OPTO4.8
VCORE
  Top 0.305: C18.2 U6.20
VEE-
  Top 0.508: OPTO1.5 57.91,34.87 57.91,43.23 OPTO3.5 | OPTO3.5
  Bottom 0.508: OPTO5.5 66.45,30.35 58.93,30.35 OPTO1.5 | OPTO1.5 | OPTO2.5 59,49 59,46.94 57.07,45.01 OPTO3.5
  Bottom 0.762: VEE-VCC+.2 68.43,82.02 65.74,79.32 65.74,71.81 66.62,70.92 68.33,70.92 OPTO4.5 68.99,68.25 65.91,65.18 65.91,53.82 64.85,52.76 62.76,52.76 OPTO2.5
VNN-  (via drill 0.3, 0.3 pad 0.81, 0.6)
  Top 0.508: OPTO7.5 4.09,7.11 VPP_VNN.2 | OPTO6.5 v28.65,17.98 | v45.24,9.07 OPTO10.5 38.79,17.93 OPTO8.5 | v61.11,11.18 59.66,9.73 v58.27,9.73
  Bottom 0.508: OPTO9.5 71.22,57.48 72.62,56.08 72.62,13.39 70.38,11.15 61.14,11.15 v61.11,11.18 | v45.24,9.07 45.36,8.94 57.48,8.94 v58.27,9.73 | OPTO7.5 5.92,13.44 20.27,13.44 OPTO6.5 | v28.65,17.98 31.85,14.78 35.43,14.78 OPTO8.5
VO1
  Top 0.508: OPTO1.7 54.28,36.32 54.28,32.54 57.1,29.72 57.1,19.61 61.8,14.91 J5.11
VO2  (via drill 0.6)
  Top 0.508: OPTO2.7 64.39,46 64.39,44.6 63.78,43.99 60.81,43.99 60.38,43.56 v60.38,21.26
  Bottom 0.508: v60.38,21.26 60.63,21.26 J5.9
VO3
  Top 0.203: J5.7 59,19.99 58.6,20.4 58.6,49.68 58.19,50.09 OPTO3.7
VO4
  Top 0.508: OPTO4.7 71.96,75.34 74.14,73.15 74.14,27.51 70.41,23.77 65.68,23.77 J5.5
VO5
  Top 0.508: OPTO5.7 71.68,35.94 71.68,28.58 68.17,25.07 J5.4
VO6
  Top 0.762: OPTO6.7 20.96,16.76 20.96,6.83 26.04,1.75 69.32,1.75 71.22,3.66 71.22,20.42 69.11,22.53 J5.6
VO7  (via drill 0.6)
  Top 0.762: v61.06,3.07 68.96,3.07 69.82,3.94 69.82,12.07 J5.12
  Bottom 0.762: OPTO7.7 17.7,3.07 v61.06,3.07
VO8  (via drill 0.61)
  Top 0.508: OPTO8.7 33.5,14.58 v34.32,13.77 | v38,13.77 41.15,13.77 v42.44,12.47 | v53.92,14.61 55.5,13.03 v57,13.03
  Bottom 0.508: v34.32,13.77 v38,13.77 | v42.44,12.47 44.58,14.61 v53.92,14.61 | v57,13.03 57.63,13.67 65.74,13.67 66.98,12.42 J5.14
VO9
  Bottom 0.635: OPTO9.7 72.03,62.56 73.74,60.86 73.74,12.27 71.58,10.11 67.26,10.11 J5.16
VO10
  Top 0.508: OPTO10.7 52.15,13.31 53.65,13.31 55.02,11.94 55.02,10.97 57.46,8.53 65.74,8.53 J5.18
VPP+  (via drill 0.61)
  Top 0.508: VPP_VNN.1 6.96,3.3 11.71,8.05 OPTO7.8 17.2,17.09 OPTO6.8 19.38,20.17 28.78,20.17 30.96,17.98 OPTO8.8 32.21,16.69 32.21,10.03 34.21,8.03 49.4,8.03 OPTO10.8 | OPTO10.8
  Top 0.635: OPTO10.8 58.27,6.07 v58.27,6.05
  Bottom 0.635: v58.27,6.05 58.29,6.02 72.39,6.02 75.26,8.89 75.26,61.42 71.58,65.1 OPTO9.8

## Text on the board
tDocu: GND | RST | 5V | 3V3 | RTS >> | CTS << | RXD << | TXD >> | SBW RST | SBW TST | Rev1.5 | 3V3 | 5V | P6.5 | GND | P3.4 | P6.0 | P3.3 | P6.1 | P1.6 | P6.2 | P6.6 | P6.3 | P3.2 | P6.4 | P2.7 | P7.0 | P4.2 | P3.6 | P4.1 | P3.5 | GND | P1.1 | P2.5 | P2.1 | GND | GND | GND | GND | P2.4 | VO5 | 5V | VO4 | 3V3 | VO6 | VO3 | P7.4 | VO2 | RST | VO1 | VO7 | P4.3 | VO8 | P4.0 | VO9 | P3.7 | VO10 | P8.2 | P8.1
